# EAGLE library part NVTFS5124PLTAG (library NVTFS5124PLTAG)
Low On-Resistance; Low Capacitance; AECQ101 Qualified and PPAP Capable; Small Footprint (3.3 x 3.3 mm); NVTFS5124PLWF Wettable Flanks Product; RoHS Compliant Source: Datasheet
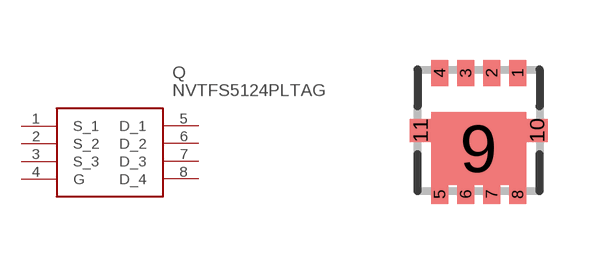
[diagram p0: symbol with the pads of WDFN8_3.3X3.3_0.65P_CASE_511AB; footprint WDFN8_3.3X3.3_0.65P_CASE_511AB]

Designator prefix Q

## NVTFS5124PLTAG (Arrow_Part_Number: NVTFS5124PLTAG; Arrow_Price-Stock: https://www.arrow.com/en/products/nvtfs5124pltag/on-semiconductor; Description: Low On-Resistance; Low Capacitance; AECQ101 Qualified and PPAP Capable; Small Footprint (3.3 x 3.3 mm); NVTFS5124PLWF Wettable Flanks Product; RoHS Compliant; Height: mm; Manufacturer_Name: onsemi; Manufacturer_Part_Number: NVTFS5124PLTAG; Mouser_Part_Number: 863-NVTFS5124PLTAG; Mouser_Price-Stock: https://www.mouser.co.uk/ProductDetail/onsemi/NVTFS5124PLTAG?qs=8%252BXDBfnGdBywpAb9wsWb%2FQ%3D%3D)  [WDFN8_3.3X3.3_0.65P_CASE_511AB]
1  S_1
2  S_2
3  S_3
4  G  in
5  D_1
6  D_2
7  D_3
8  D_4

## Footprint WDFN8_3.3X3.3_0.65P_CASE_511AB (pad centres in mm)
WDFN8 3.3x3.3, 0.65P CASE 511AB ISSUE D_1
smd 0.42 x 0.66: 1 0.975,1.435; 2 0.325,1.435; 3 -0.325,1.435; 4 -0.975,1.435
smd 0.42 x 0.47: 5 -0.975,-1.6; 6 -0.325,-1.6; 7 0.325,-1.6; 8 0.975,-1.6
smd 2.37 x 1.83: 9 0,-0.45
smd 0.545 x 0.57: 10 1.458,0; 11 -1.458,0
